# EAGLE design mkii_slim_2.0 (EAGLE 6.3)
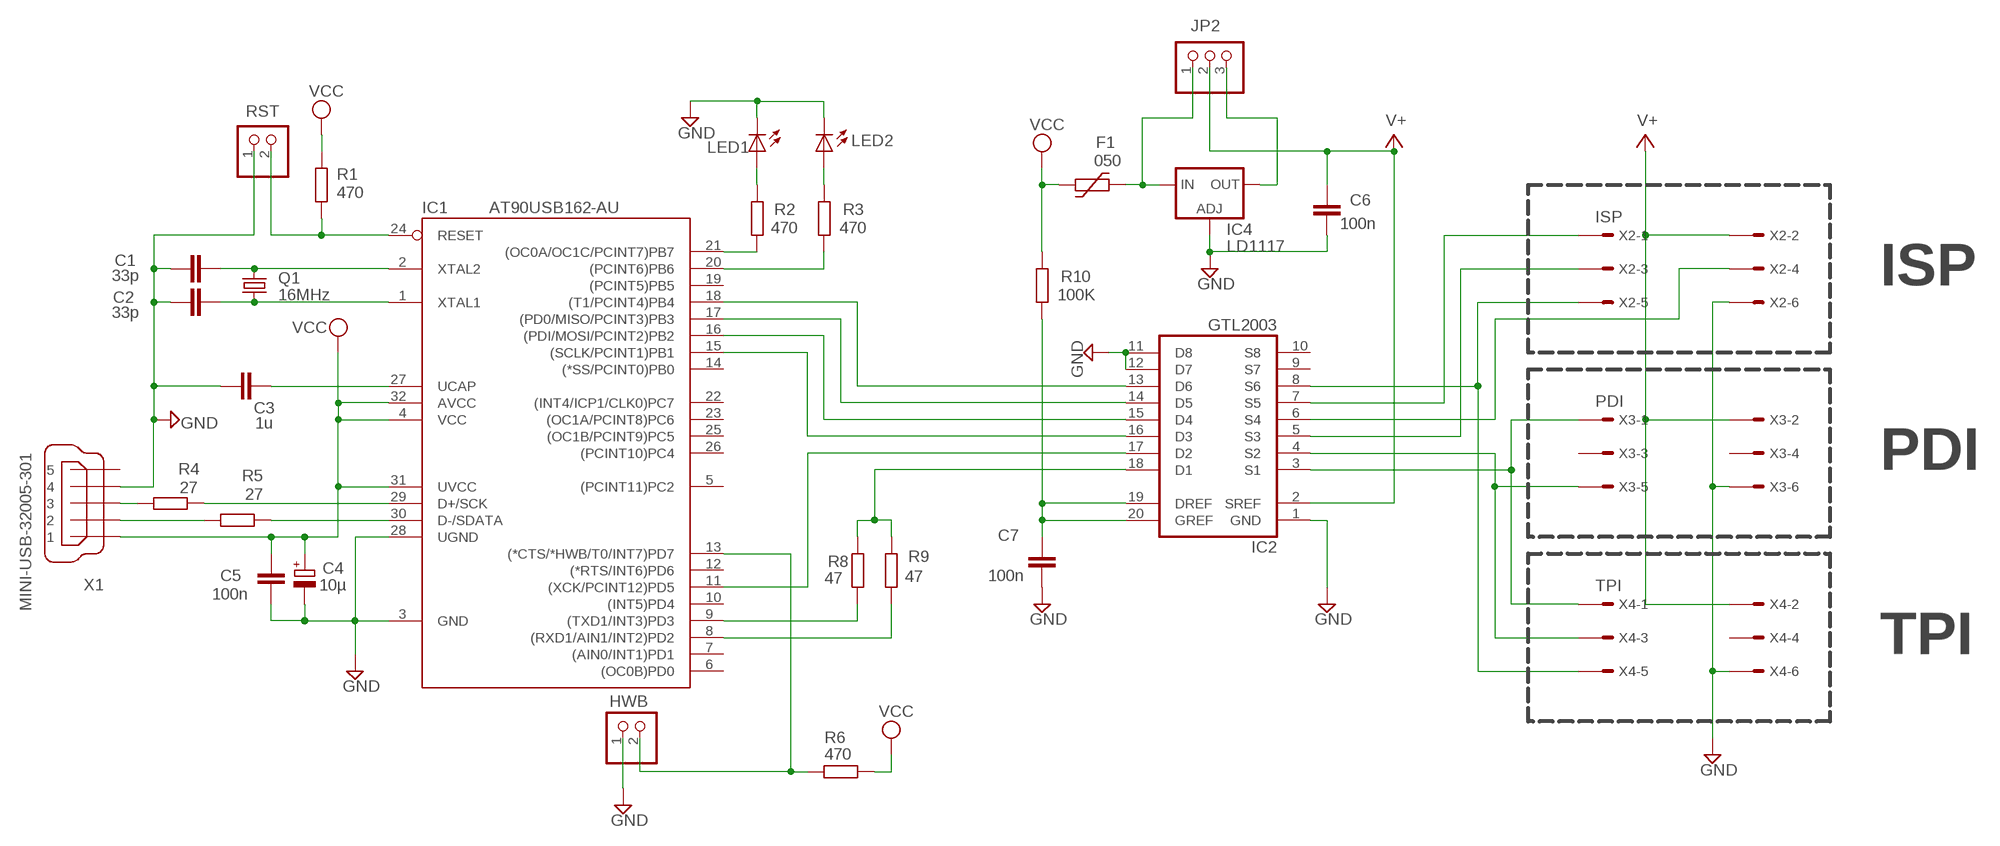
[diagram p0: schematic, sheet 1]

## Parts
C1  33p  C-EUC0805  [C0805]
C2  33p  C-EUC0805  [C0805]
C3  1u  C-EUC1206  [C1206]
C4  10µ  CPOL-EUCT6032  [CT6032]
C5  100n  C-EUC0805  [C0805]
C6  100n  C-EUC0805  [C0805]
C7  100n  C-EUC0805  [C0805]
F1  050  1812L  [1812L]
HWB  PINHD-1X02_2.54-S  [1X02-S]
IC1  AT90USB162-AU  [TQFP32-08]
IC2  GTL2003  [TSSOP20]
IC4  LD1117  LD117AS33TR  [SOT223]
JP2  PINHD-1X03_2.54  [1X03]
LED1  LEDCHIPLED_0805  [CHIPLED_0805]
LED2  LEDCHIPLED_0805  [CHIPLED_0805]
Q1  16MHz  CRYSTALSM49  [SM49]
R1  470  R-EU_M0805  [M0805]
R2  470  R-EU_M0805  [M0805]
R3  470  R-EU_M0805  [M0805]
R4  27  R-EU_M0805  [M0805]
R5  27  R-EU_M1206  [M1206]
R6  470  R-EU_M0805  [M0805]
R8  47  R-EU_M0805  [M0805]
R9  47  R-EU_M0805  [M0805]
R10  100K  R-EU_M0805  [M0805]
RST  PINHD-1X02_2.54-S  [1X02-S]
X1  MINI-USB-32005-301  [32005-301]
X2  ISP  057-006-1  [057-006-1]
X3  PDI  057-006-1  [057-006-1]
X4  TPI  057-006-1  [057-006-1]

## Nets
GND: C1.1 C2.1 C3.1 C4.- C5.1 C6.1 C7.1 HWB.1 IC1.3(GND) IC1.28(UGND) IC2.1(GND) IC2.11(D8) IC2.12(D7) IC4.1(ADJ) LED1.C LED2.C RST.1 X1.4 X2.6 X3.6 X4.6
N$1: R4.2 X1.3
N$2: R5.2 X1.2
N$3: IC1.29(D+/SCK) R4.1
N$4: C3.2 IC1.27(UCAP)
N$5: C1.2 IC1.2(XTAL2) Q1.2
N$6: C2.2 IC1.1(XTAL1) Q1.1
N$7: IC1.30(D-/SDATA) R5.1
N$8: IC1.24(RESET) R1.1 RST.2
N$9: IC1.9((TXD1/INT3)PD3) R8.2
N$10: IC1.21((OC0A/OC1C/PCINT7)PB7) R2.2
N$11: IC1.20((PCINT6)PB6) R3.2
N$12: LED1.A R2.1
N$13: LED2.A R3.1
N$14: HWB.2 IC1.13((*CTS/*HWB/T0/INT7)PD7) R6.1
N$15: C7.2 IC2.19(DREF) IC2.20(GREF) R10.2
N$16: IC1.18((T1/PCINT4)PB4) IC2.13(D6)
N$17: IC1.17((PD0/MISO/PCINT3)PB3) IC2.14(D5)
N$18: IC1.16((PDI/MOSI/PCINT2)PB2) IC2.15(D4)
N$19: IC1.15((SCLK/PCINT1)PB1) IC2.16(D3)
N$20: IC1.11((XCK/PCINT12)PD5) IC2.17(D2)
N$21: IC2.18(D1) R8.1 R9.1
N$22: F1.P$2 IC4.3(IN) JP2.1
N$23: IC4.4(OUT) JP2.3
N$25: IC2.3(S1) X3.1 X4.1
N$26: IC2.4(S2) X3.5 X4.3
N$27: IC2.8(S6) X2.5 X4.5
N$28: IC2.7(S5) X2.1
N$29: IC2.6(S4) X2.4
N$30: IC2.5(S3) X2.3
N$31: IC1.8((RXD1/AIN1/INT2)PD2) R9.2
V+: C6.2 IC2.2(SREF) JP2.2 X2.2 X3.2 X4.2
VCC: C4.+ C5.2 F1.P$1 IC1.4(VCC) IC1.31(UVCC) IC1.32(AVCC) R1.2 R6.2 R10.1 X1.1
Unconnected: IC1.5((PCINT11)PC2) IC1.6((OC0B)PD0) IC1.7((AIN0/INT1)PD1) IC1.10((INT5)PD4) IC1.12((*RTS/INT6)PD6) IC1.14((*SS/PCINT0)PB0) IC1.19((PCINT5)PB5) IC1.22((INT4/ICP1/CLK0)PC7) IC1.23((OC1A/PCINT8)PC6) IC1.25((OC1B/PCINT9)PC5) IC1.26((PCINT10)PC4) IC2.9(S7) IC2.10(S8) X1.5 X3.3 X3.4 X4.4

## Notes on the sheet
- ISP
- PDI
- TPI

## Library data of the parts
C1-C3 C5-C7 = rcl:C-EU: CAPACITOR, European symbol
C4 = rcl:CPOL-EU: POLARIZED CAPACITOR, European symbol
F1 = ptc-littlefuse:1812L
HWB RST = pinhead-2:PINHD-1X02: PIN HEADER
IC1 = at90usb:AT90USB162-*
IC2 = manekinen_diy:GTL2003: "8-bit bidirectional low voltage translator"
IC4 = v-reg:LD117A?*: Low drop fixed and adjustable positive voltage regulators 1 A Source: http://www.st.com/stonline/products/literature/ds/7194/ld1117axx.pdf
JP2 = pinhead-2:PINHD-1X03: PIN HEADER
LED1 LED2 = led:LED: LED
Q1 = crystal:CRYSTAL: CRYSTAL
R1-R6 R8-R10 = rcl:R-EU_: RESISTOR, European symbol
X1 = con-cypressindustries:MINI-USB-: MINI USB-B Conector Source: www.cypressindustries.com
X2-X4 = con-panduit:057-006-: CONNECTOR 6-pin series 057 contact pc board low profile headers

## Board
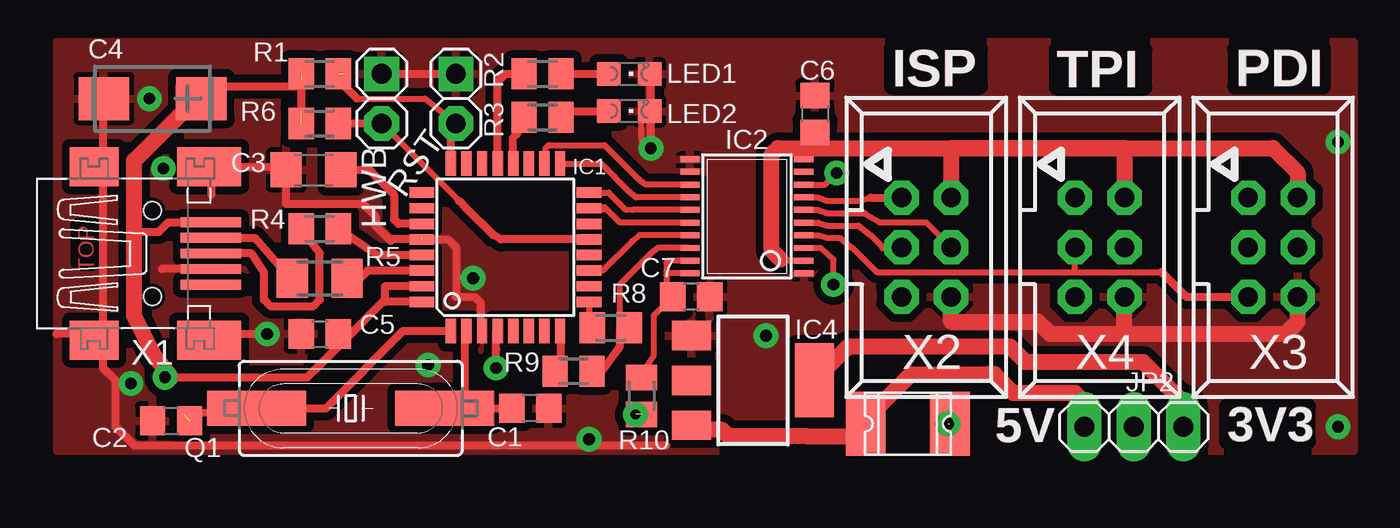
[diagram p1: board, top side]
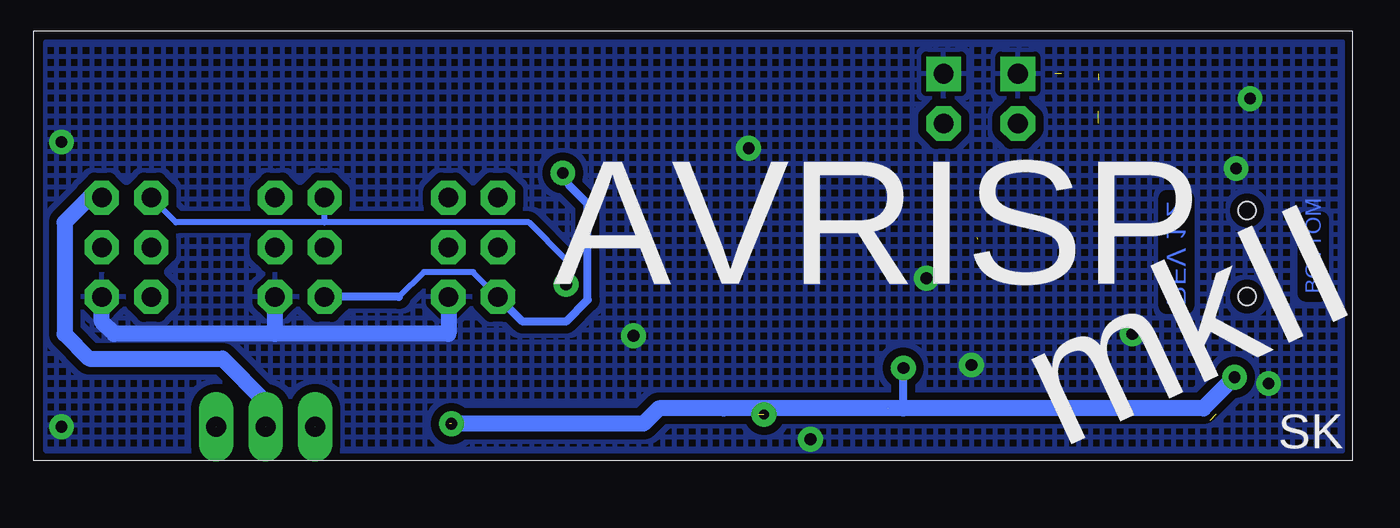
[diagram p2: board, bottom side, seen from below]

No outline drawn. Coordinates in mm, seen from the top.
Copper layers (1*16): Top 0.035mm / dielectric 1.5mm / Bottom 0.035mm
Design rules "default *": minimum track width 10mil, minimum drill 24mil, track to track 16mil, track to pad 16mil, pad to pad 16mil, via to via 16mil, smd to smd 16mil, copper to edge 8mil, drill to drill 8mil, minimum pad ring 15mil, minimum via ring 8mil, stop-mask expansion 4mil, vias tented up to drill 32mil, thermal gap 10mil

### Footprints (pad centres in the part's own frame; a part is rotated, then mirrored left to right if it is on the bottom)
C0805 = smd 1.3 x 1.5: 1 -0.95,0; 2 0.95,0
C1206 = smd 1.6 x 1.8: 1 -1.4,0; 2 1.4,0
CT6032 = smd 2.6 x 2.2: + -2.5,0; - 2.5,0
1812L = smd 2.03 x 3.3: P$1 -2.16,0; P$2 2.16,0
1X02-S = drill 1.016 square: 1 -1.27,0 | drill 1.016 octagon: 2 1.27,0
TQFP32-08 = smd 1.27 x 0.533: 1 -4.293,2.8; 2 -4.293,2; 3 -4.293,1.2; 4 -4.293,0.4; 5 -4.293,-0.4; 6 -4.293,-1.2; 7 -4.293,-2; 8 -4.293,-2.8; 17 4.293,-2.8; 18 4.293,-2; 19 4.293,-1.2; 20 4.293,-0.4; 21 4.293,0.4; 22 4.293,1.2; 23 4.293,2; 24 4.293,2.8 | smd 0.533 x 1.27: 9 -2.8,-4.293; 10 -2,-4.293; 11 -1.2,-4.293; 12 -0.4,-4.293; 13 0.4,-4.293; 14 1.2,-4.293; 15 2,-4.293; 16 2.8,-4.293; 25 2.8,4.293; 26 2,4.293; 27 1.2,4.293; 28 0.4,4.293; 29 -0.4,4.293; 30 -1.2,4.293; 31 -2,4.293; 32 -2.8,4.293
TSSOP20 = smd 0.991 x 0.305: 1 -2.918,2.925; 2 -2.918,2.275; 3 -2.918,1.625; 4 -2.918,0.975; 5 -2.918,0.325; 6 -2.918,-0.325; 7 -2.918,-0.975; 8 -2.918,-1.625; 9 -2.918,-2.275; 10 -2.918,-2.925; 11 2.918,-2.925; 12 2.918,-2.275; 13 2.918,-1.625; 14 2.918,-0.975; 15 2.918,-0.325; 16 2.918,0.325; 17 2.918,0.975; 18 2.918,1.625; 19 2.918,2.275; 20 2.918,2.925
SOT223 = smd 1.5 x 2: 1 -2.3,-3.15; 2 0,-3.15; 3 2.3,-3.15 | smd 3.8 x 2: 4 0,3.15
1X03 = drill 1.016 long: 1 -2.54,0; 2 0,0; 3 2.54,0
CHIPLED_0805 = smd 1.2 x 1.2: A 0,-1.05; C 0,1.05
SM49 = smd 5.08 x 1.778: 1 -4.826,0; 2 4.826,0
M0805 = smd 1.3 x 1.6: 1 -0.95,0; 2 0.95,0
M1206 = smd 1.6 x 2: 1 -1.4,0; 2 1.4,0
32005-301 = smd 3.1 x 0.5: 1 3,1.6; 2 3,0.8; 3 3,0; 4 3,-0.8; 5 3,-1.6 | smd 2.5 x 2: M1 -3,-4.45; M2 -3,4.45 | smd 3.3 x 2: M3 2.9,4.45; M4 2.9,-4.45 | hole 0.9: 0,2.2; 0,-2.2
057-006-1 = drill 1 octagon: 1 -2.54,-1.27; 2 -2.54,1.27; 3 0,-1.27; 4 0,1.27; 5 2.54,-1.27; 6 2.54,1.27

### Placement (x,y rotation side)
C1  24.77,2.7 180 top
C2  6.35,2.06 0 top
C3  13.65,14.92 0 top
C4  5.4,18.57 180 top
C5  13.97,6.51 0 top
C6  39.37,17.78 270 top
C7  33.02,8.41 180 top
F1  44.13,1.9 180 top
HWB  17.14,18.57 270 top
IC1  23.5,10.95 90 top
IC2  35.88,12.54 180 top
IC4  36.2,4.13 270 top
JP2  55.72,1.75 0 top
LED1  29.84,19.84 270 top
LED2  29.84,17.94 270 top
Q1  15.56,2.7 0 top
R1  13.97,19.84 180 top
R2  25.4,19.84 180 top
R3  25.4,17.62 180 top
R4  13.97,11.91 180 top
R5  13.97,9.37 180 top
R6  13.97,17.3 180 top
R8  28.89,6.83 180 top
R9  26.99,4.6 180 top
R10  30.48,3.33 90 top
RST  20.95,18.57 270 top
X1  5.4,10.64 0 top
X2  45.09,10.95 270 top
X3  62.87,10.95 270 top
X4  53.98,10.95 270 top

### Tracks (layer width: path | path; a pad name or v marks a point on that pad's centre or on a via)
GND  (via drill 0.6 pad 1.27)  (1 unrouted)
  Top 0.305: IC1.3 22.23,6.66 22.23,6.67 | v30.96,16.03 30.64,16.03 30.48,16.51 30.48,17.52 LED2.C | X1.4
  Top 0.406: 19.21,11.27 19.21,11.43 | 22.23,6.67 22.23,8.1 21.91,8.41 20.95,8.41 20.95,10.95 20.55,11.35 IC1.28 17.7,11.35 17.62,11.27 16.83,12.06 16.83,12.54 16.19,13.18 12.22,13.18 12.22,15.08 8.41,15.08 | 31.75,0.79 4.45,0.79 3.49,1.75 3.49,4.13 2.86,4.76 2.86,6.51 | 2.86,6.51 2.86,15.4 | 3.81,18.89 2.86,17.94 2.86,15.4 | 30.96,15.88 v30.96,16.03 30.96,19.84 | 8.57,6.51 v11.27,6.51 | HWB.1 RST.1 | 8.57,9.84 X1.4 5.87,9.84 | 6.99,15.08 8.41,15.08 | 8.41,15.08 8.41,13.65 | 2.86,6.51 0.48,6.51 | 2.86,15.4 2.7,15.4
  Top 0.813: 55.24,6.51 51.44,6.51 50.8,7.14 46.35,7.14 X2.6 | 55.24,6.51 63.5,6.51 64.14,7.14 X3.6 | 55.24,6.51 X4.6
  Bottom 0.813: X2.6 46.35,6.51 55.24,6.51 | 55.24,6.51 63.5,6.51 64.14,7.14 X3.6 | 55.24,6.51 X4.6
  other vias: 4.29,3.97 5.95,14.99 21.84,9.37 36.85,6.41 66.2,1.75 27.78,1.11 19.53,4.92 5.24,18.57 66.2,16.35
  pour Top: 0.5,21.5 67,21.5 67,0.5 0.5,0.5
  pour Bottom (isolate 0.406, hatched): 0.5,21.5 0.5,0.5 67,0.5 67,21.5
N$1
  Top 0.305: 8.89,10.64 X1.3
  Top 0.406: 8.89,10.64 10.48,10.64 11.11,9.68 11.11,8.26 11.43,7.94 13.65,7.94 13.97,8.26 13.97,10.64 R4.2
N$2
  Top 0.305: X1.2 8.57,11.44 8.57,11.43 | 12.7,9.05 12.7,9.24 R5.2
  Top 0.406: 8.57,11.43 10.64,11.43 12.7,9.05 12.38,9.05
N$3
  Top 0.406: IC1.29 16.91,10.55 R4.1
N$4  (1 unrouted)
  Top 0.406: 15.08,14.92 16.51,14.92 17.78,13.65 17.78,12.38 18.01,12.15 IC1.27
N$5  (1 unrouted)
  Top 0.305: 21.43,6.67 IC1.2 | 21.43,2.7 Q1.2
  Top 0.406: 21.43,6.67 21.43,2.7 C1.2
N$6  (1 unrouted)
  Top 0.305: IC1.1 20.64,6.66 20.64,6.67
  Top 0.406: 20.64,6.67 18.26,6.67 14.29,2.7 Q1.1 6.99,2.38
N$7
  Top 0.406: IC1.30 16.42,9.75 15.88,9.21 15.08,9.21 R5.1
N$8  (1 unrouted)
  Top 0.305: 15.88,18.57 19.37,18.57 RST.2 20.7,17.04
  Top 0.406: 15.88,18.57 15.24,19.21 15.24,19.84 | IC1.24 20.7,17.04
N$9
  Top 0.305: 27.78,8.1 27.78,6.67 R8.2 | IC1.9 27.88,8.15 27.94,8.1
  Top 0.406: 28.1,8.1 27.94,8.1 27.78,8.1
N$10
  Top 0.305: R2.2
  Top 0.406: R2.2 23.5,19.84 23.34,19.68 23.09,19.44 IC1.21
N$11
  Top 0.406: IC1.20 23.89,16.59 24.13,16.83 24.13,17.62 R3.2
N$12
  Top 0.305: LED1.A 28.73,19.84 | R2.1
  Top 0.406: R2.1 28.73,19.84
N$13
  Top 0.305: LED2.A 28.73,17.94 | 26.35,17.94 R3.1
  Top 0.406: 26.35,17.94 28.73,17.94
N$14  (1 unrouted)
  Top 0.305: HWB.2 21.11,13.34
  Top 0.406: 21.11,13.34 21.43,13.02 22.86,11.59 23.26,11.35 IC1.13 | R6.1 HWB.2
N$15
  Top 0.305: IC2.19 31.86,10.27 31.75,10.16 31.75,9.71 31.84,9.62 | IC2.20 31.84,9.62 | 31.84,9.62 31.75,9.53 31.75,8.73 C7.2 31.11,7.46 31.11,5.4 30.48,4.45 R10.2
N$16
  Top 0.305: 25.56,15.24 25.56,16.03 25.72,16.19 28.57,16.19 30.32,14.45 30.68,14.17 IC2.13
  Top 0.406: 25.56,15.08 25.56,15.24 25.55,15.25 IC1.18
N$17
  Top 0.305: IC1.17 28.42,15.24 29.84,13.81 30.18,13.52 IC2.14
  Top 0.406: IC1.17
N$18
  Top 0.305: IC1.16 28.79,13.75 29.69,12.86 30.01,12.87 IC2.15
N$19
  Top 0.305: 28.51,12.95 28.57,13.02 29.38,12.22 IC2.16
  Top 0.406: IC1.15 28.51,12.95
N$20
  Top 0.305: IC1.11 28.49,9.75 30,11.27 30.34,11.57 IC2.17
N$21
  Top 0.305: R8.1 29.52,6.51 29.37,6.67 29.37,9.05 30.96,10.64 31.31,10.92 IC2.18
  Top 0.406: 29.37,6.67 29.37,6.51 29.37,5.87 28.42,4.6 28.26,4.6 | R9.1 28.26,4.6 | R9.1 | R9.1 28.26,4.6
N$22  (1 unrouted)
  Top 0.305: F1.P$2 41.75,1.91 41.2,1.35 | 38.89,1.27 38.91,1.27
  Top 0.813: JP2.1 53.18,3.02 52.7,3.49 49.53,3.49 48.58,4.45 48.26,4.45 44.29,4.45 41.2,1.35 41.12,1.27 38.89,1.27 34.92,1.27 34.61,1.59 33.28,1.59 IC4.3
N$23  (1 unrouted)
  Top 0.813: JP2.3 58.26,3.02 56.2,5.08 50.16,5.08 49.37,5.87 41.09,5.87 IC4.4
N$25  (via drill 0.6 pad 1.27)
  Top 0.305: v40.32,9.05 40.32,10.32 39.65,10.92 IC2.3
  Bottom 0.305: 52.7,12.22 X4.1 | 52.7,12.22 42.23,12.22 40.32,10.32 v40.32,9.05 | 52.7,12.22 60.33,12.22 X3.1
N$26
  Top 0.305: 52.7,9.68 57.15,9.68 | 52.7,9.68 X4.3 | 52.7,9.68 42.55,9.68 41.27,10.95 41.25,10.93 40.64,11.43 40.01,11.43 39.55,11.57 IC2.4
  Top 0.406: X3.5 58.42,8.41 57.15,9.68
N$27  (via drill 0.6 pad 1.27)
  Top 0.305: IC2.8 39.88,14.17 40.16,14.45
  Top 0.406: 40.16,14.45 v40.48,14.76
  Bottom 0.305: X2.5 45.09,9.68 47.62,9.68 48.9,8.41
  Bottom 0.406: v40.48,14.76 40.16,14.13 39.21,13.18 39.21,8.26 40.32,7.14 42.55,7.14 X2.5 | 48.9,8.41 X4.5
N$28
  Top 0.305: IC2.7 39.51,13.52 40.01,13.34 41.59,13.34 42.23,13.49
  Top 0.406: 42.23,13.49 | 42.23,13.49 X2.1
N$29
  Top 0.305: X2.4 45.08,12.23 42.7,12.23 41.91,12.7 40.01,12.7 39.52,12.87 IC2.6
N$30
  Top 0.305: 42.86,10.95 42.23,11.59 42.22,11.58 41.59,12.06 40.01,12.06 39.54,12.22 IC2.5
  Top 0.406: 42.86,10.95 X2.3
N$31
  Top 0.305: 26.35,6.67 IC1.8
  Top 0.406: 26.35,6.67 26.35,4.6 R9.2
V+  (1 unrouted)
  Top 0.305: IC2.2 37.68,10.27 37.62,10.32 | C6.2 39.37,16.03
  Top 0.813: 55.24,16.03 39.53,16.03 39.37,16.03 37.47,16.03 37.15,15.72 37.15,10.79 37.62,10.32 | 55.24,16.03 62.87,16.03 64.14,14.76 X3.2 | 55.24,16.03 46.35,16.03 X2.2 | 55.24,16.03 X4.2
  Bottom 0.813: JP2.2 55.72,3.02 57.94,5.24 64.77,5.24 66.04,6.51 66.04,12.22 64.77,13.49 X3.2
VCC  (via drill 0.5 pad 1.27, 0.6 pad 1.27)  (5 unrouted)
  Top 0.305: 23.02,6.67 23.09,6.67 IC1.4 | 23.02,4.6 v23.02,4.76 | v23.02,4.76 | 8.57,12.22 8.41,12.22 X1.1
  Top 0.406: 6.35,4.29 13.34,4.29 15.24,6.19 | 15.24,6.19 17.3,8.26 | 5.4,5.56 4.6,7.14 4.45,7.46 | 4.45,11.75 5.71,11.75 6.19,12.22 6.99,12.22 8.57,12.22 | 23.02,4.6 23.02,5.71 23.02,6.67 | 6.99,19.21 7.62,19.21 | 7.62,19.21 13.02,19.21 | 13.02,19.21 13.02,19.53 | 13.02,19.21 13.02,17.94 | 13.65,4.6 14.92,5.87 C5.2 15.24,6.19 | IC1.32 17.3,8.15 17.3,8.26 | IC1.31 17.3,8.95 17.3,8.26 | C4.+ 7.94,18.57 7.94,18.41 7.62,18.41 7.62,19.21
  Top 0.813: v6.03,4.29 6.35,4.29 5.71,5.08 5.4,5.56 4.45,7.46 4.45,11.75 4.45,15.4 6.99,17.94 6.99,19.21
  Bottom 0.406: 23.02,2.7 v23.02,4.76 | 32.23,2.7 | 32.23,2.7 30.16,2.7 v30.16,2.38
  Bottom 0.813: v6.03,4.29 7.62,2.7 23.02,2.7 32.23,2.7 35.56,2.7 36.35,1.91 v46.2,1.91

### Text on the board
Top: ISP | TPI | PDI | TOP | 5V | 3V3
Bottom: BOTTOM | REV 1.2
tNames: ISP | TPI | PDI | 5V | 3V3
bNames: AVRISP | SK | mkII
